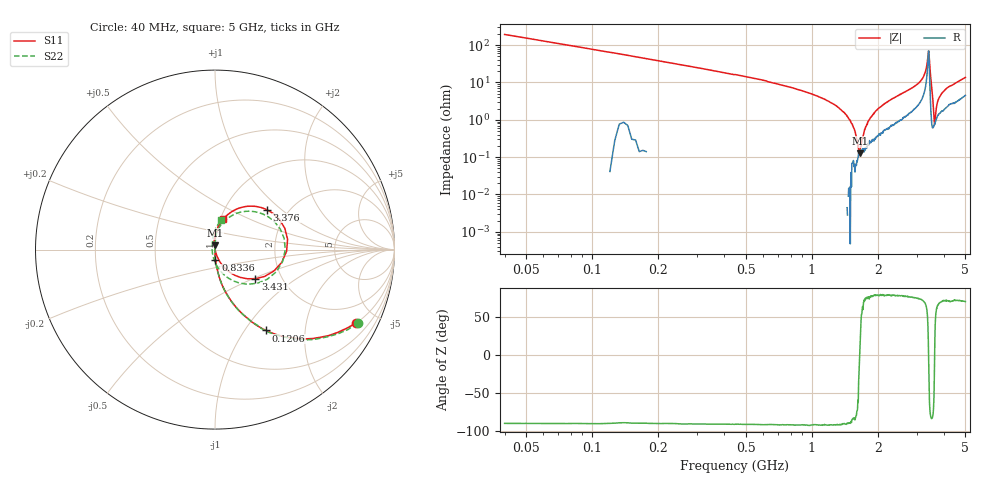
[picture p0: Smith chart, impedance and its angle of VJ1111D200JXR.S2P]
! VJ1111D200JXR
! DATE 02/16/2022  10:13
! CAPACITORS MOUNTED IN SERIES ON 25 MIL THICK MICROSTRIP SUBSTRATE
# GHz  S  MA  R  50.00
!  FREQ  S11M  S11A  S21M  S21A  S12M  S12A  S22M  S22A
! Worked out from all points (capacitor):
!   801 points, 40 MHz to 5 GHz, reference 50 ohm
!   read as one part in series: C = 20.5 pF near 64.8 MHz
!   lowest |Z| = 127 mohm at 1.652 GHz (marker M1)
!   series resonance near 1.651 GHz, so ESL is about 450 pH
!   S11 on the Smith chart (normalised r, x): 40 MHz: 1.01, -3.86; 120.6 MHz: 1.00, -1.26; 833.6 MHz: 1.00, -0.12; 3.376 GHz: 1.56, +0.80; 3.431 GHz: 1.47, -0.52; 5 GHz: 1.02, +0.36
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0.04  0.8869 -27.4  0.4612 62.6  0.4599 62.6  0.894 -27.3
0.1206  0.5336 -57.6  0.834 32.5  0.8524 32.9  0.542 -57.6
0.3004  0.239 -76.2  0.9712 14.3  0.978 14.1  0.2405 -76.5
0.8336  0.05875 -87.9  0.9986 4.6  1.004 4.5  0.05734 -87.7
0.8708  0.0521 -87.8  0.9994 4.4  1.004 4.3  0.05174 -87.7
1.2304  0.01118 -92.4  0.9981 2.7  1.003 2.5  0.01127 -93.4
1.2924  0.006284 -93.6  0.9978 2.5  1.004 2.3  0.005418 -99.0
1.3482  0.0007678 -164.4  0.9979 2.2  1.003 2.1  0.0008544 -154.1
1.466  0.008854 98.1  0.9961 1.9  1.002 1.7  0.009498 94.9
1.652  0.02328 90.9  0.9947 1.4  1 1.3  0.02319 89.7
1.6954  0.02599 91.0  0.9941 1.3  0.9996 1.1  0.02633 90.2
2.52  0.07904 86.1  0.9795 -0.6  0.9853 -0.8  0.08007 85.8
3.1586  0.1489 78.2  0.9447 -3.8  0.9504 -3.9  0.1466 75.8
3.3508  0.3002 53.5  0.8006 -10.2  0.8051 -10.3  0.2884 47.9
3.3756  0.3653 37.6  0.6884 -9.7  0.6922 -9.9  0.3505 31.0
3.4314  0.2778 -35.7  0.8085 19.0  0.814 18.8  0.2662 -46.5
3.5244  0.01489 -73.3  0.9765 6.0  0.9818 5.9  0.02195 -131.6
3.543  0.002905 95.8  0.9767 5.1  0.9824 5.0  0.01615 177.7
3.5988  0.03933 97.2  0.9752 3.3  0.9806 3.1  0.03686 113.3
3.698  0.07073 92.9  0.969 1.6  0.9733 1.4  0.06082 100.1
4.1754  0.1237 82.3  0.9563 -1.0  0.9614 -1.1  0.1089 84.4
5  0.1753 76.2  0.9245 -3.9  0.9298 -4.0  0.1671 77.7
